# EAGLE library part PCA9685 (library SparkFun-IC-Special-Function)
16-channel 12-bit PWM I2C interface Internal Oscillator 40Hz to 1kHz Can be totem pole or open collector 2.3V to 5.5V SparkFun Products SparkFun Block for Intel® Edison - PWM (DEV-13042) PROTO: IC-12240 PROD_ID: IC-12271
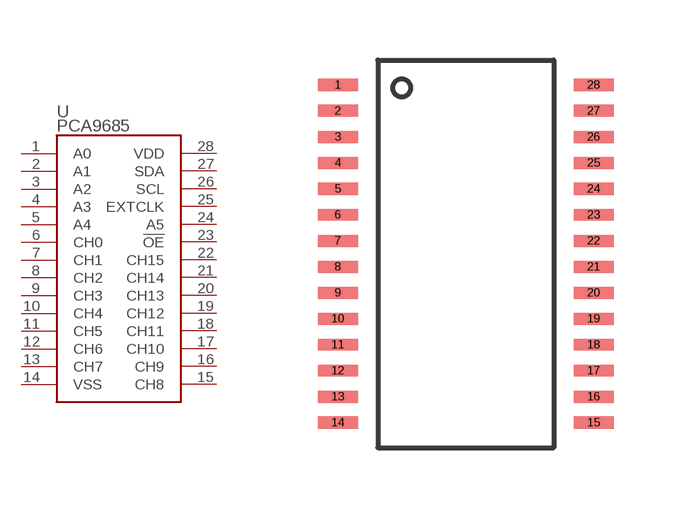
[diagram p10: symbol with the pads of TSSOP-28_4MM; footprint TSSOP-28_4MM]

Designator prefix U

## PCA9685 (PROD_ID: IC-12271; VALUE: PCA9685)  [TSSOP-28_4MM]
1  A0
2  A1
3  A2
4  A3
5  A4
6  CH0
7  CH1
8  CH2
9  CH3
10  CH4
11  CH5
12  CH6
13  CH7
14  VSS
15  CH8
16  CH9
17  CH10
18  CH11
19  CH12
20  CH13
21  CH14
22  CH15
23  !OE
24  A5
25  EXTCLK
26  SCL
27  SDA
28  VDD

## Footprint TSSOP-28_4MM (pad centres in mm)
smd 1 x 0.3: 1 -3.2,4.225; 2 -3.2,3.575; 3 -3.2,2.925; 4 -3.2,2.275; 5 -3.2,1.625; 6 -3.2,0.975; 7 -3.2,0.325; 8 -3.2,-0.325; 9 -3.2,-0.975; 10 -3.2,-1.625; 11 -3.2,-2.275; 12 -3.2,-2.925; 13 -3.2,-3.575; 14 -3.2,-4.225; 15 3.2,-4.225; 16 3.2,-3.575; 17 3.2,-2.925; 18 3.2,-2.275; 19 3.2,-1.625; 20 3.2,-0.975; 21 3.2,-0.325; 22 3.2,0.325; 23 3.2,0.975; 24 3.2,1.625; 25 3.2,2.275; 26 3.2,2.925; 27 3.2,3.575; 28 3.2,4.225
